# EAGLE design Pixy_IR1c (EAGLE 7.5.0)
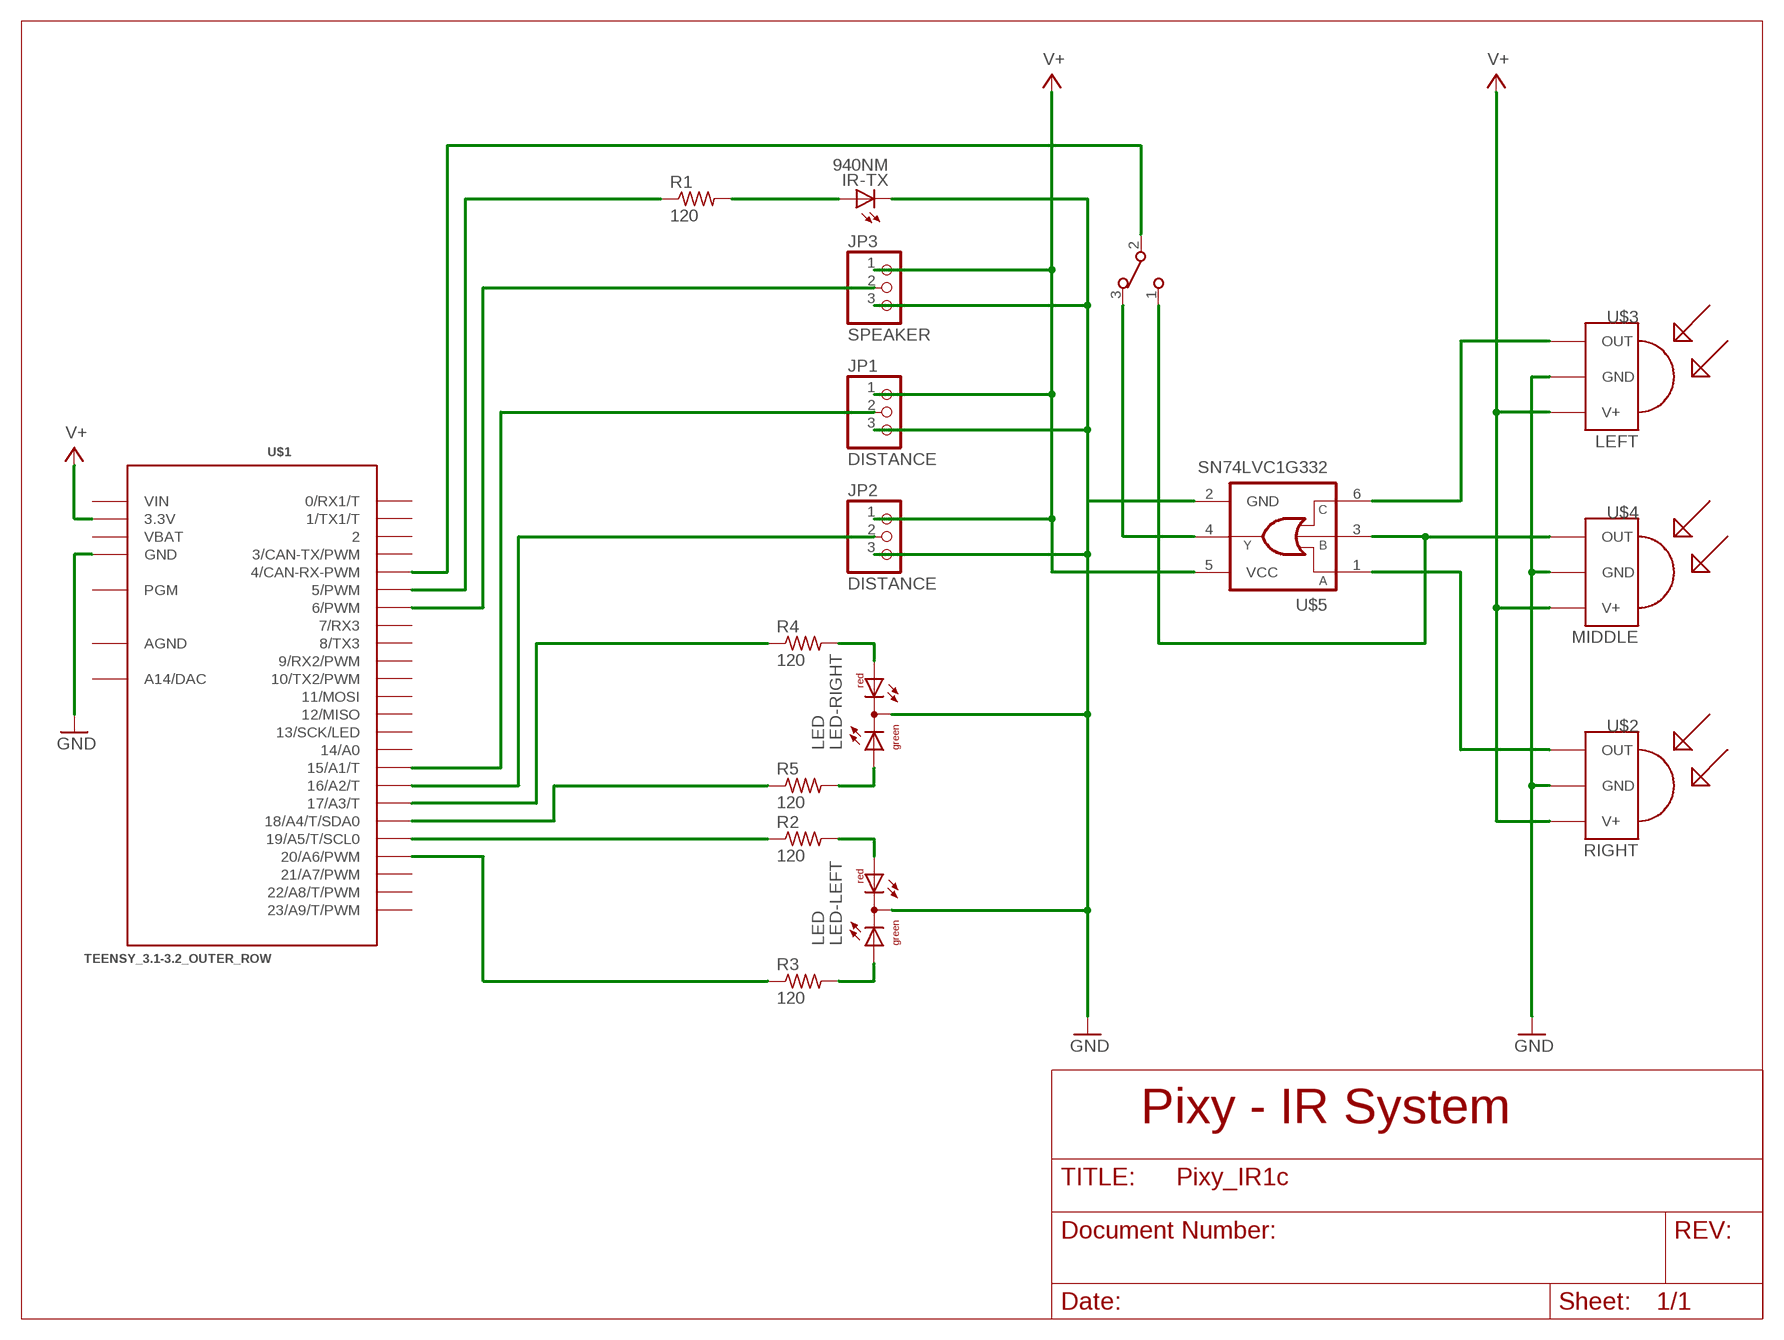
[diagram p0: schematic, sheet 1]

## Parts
IR-TX  940NM  LED5MM  [LED5MM]
JP1  DISTANCE  PINHD-1X3  [1X03]
JP2  DISTANCE  PINHD-1X3  [1X03]
JP3  SPEAKER  PINHD-1X3  [1X03]
LED-LEFT  LED  DUOLED-RG-C  [DUOLED-C-5MM]
LED-RIGHT  LED  DUOLED-RG-C  [DUOLED-C-5MM]
R1  120  R-US_R1206  [R1206]
R2  120  R-US_R1206  [R1206]
R3  120  R-US_R1206  [R1206]
R4  120  R-US_R1206  [R1206]
R5  120  R-US_R1206  [R1206]
SW1  CAS-120CAS-120B1  [CAS-120B1]
U$1  TEENSY_3.1-3.2_OUTER_ROW  [TEENSY_3.0-3.2&LC_OUTER_ROW]
U$2  RIGHT  TSOP3X  [TSOP18XX]
U$3  LEFT  TSOP3X  [TSOP18XX]
U$4  MIDDLE  TSOP3X  [TSOP18XX]
U$5  SN74LVC1G332  [SC70-6]

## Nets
GND: IR-TX.K(C) JP1.3 JP2.3 JP3.3 LED-LEFT.C LED-RIGHT.C U$1.GND U$1.GND1(GND) U$2.GND U$3.GND U$4.GND U$5.2(GND)
N$1: R2.1 U$1.19/A5(19/A5/T/SCL0)
N$2: R5.1 U$1.18/A4(18/A4/T/SDA0)
N$3: LED-RIGHT.AR R4.2
N$4: LED-RIGHT.AX(AG) R5.2
N$5: LED-LEFT.AR R2.2
N$6: LED-LEFT.AX(AG) R3.2
N$7: JP3.2 U$1.6(6/PWM)
N$8: R1.1 U$1.5(5/PWM)
N$9: R4.1 U$1.17/A3(17/A3/T)
N$10: R3.1 U$1.20/A6(20/A6/PWM)
N$11: JP1.2 U$1.15/A1(15/A1/T)
N$12: IR-TX.A R1.2
N$13: JP2.2 U$1.16/A2(16/A2/T)
N$14: SW1.2 U$1.4(4/CAN-RX-PWM)
N$15: SW1.3 U$5.4(Y)
N$16: SW1.1 U$4.OUT U$5.3(B)
N$17: U$3.OUT U$5.6(C)
N$18: U$2.OUT U$5.1(A)
V+: JP1.1 JP2.1 JP3.1 U$1.3.3V U$1.3.3V1(3.3V) U$2.VCC(V+) U$3.VCC(V+) U$4.VCC(V+) U$5.5(VCC)
Unconnected: U$1.0(0/RX1/T) U$1.1(1/TX1/T) U$1.2 U$1.3(3/CAN-TX/PWM) U$1.7(7/RX3) U$1.8(8/TX3) U$1.9(9/RX2/PWM) U$1.10(10/TX2/PWM) U$1.11(11/MOSI) U$1.12(12/MISO) U$1.13(13/SCK/LED) U$1.14/A0 U$1.21/A7(21/A7/PWM) U$1.22/A8(22/A8/T/PWM) U$1.23/A9(23/A9/T/PWM) U$1.PGM U$1.RESET/DAC(A14/DAC)

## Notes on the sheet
- Pixy - IR System

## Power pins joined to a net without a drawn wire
AGND: U$1.AGND
VBAT: U$1.VBAT
VIN: U$1.VIN

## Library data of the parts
IR-TX = led:LED: LED
JP1-JP3 = pinhead:PINHD-1X3: PIN HEADER
LED-LEFT LED-RIGHT = led:DUOLED-RG-C: DUO LED 2 colors (red/green), 5 mm, round, common Cathode www.ligitek.com or other producers.
R1-R5 = resistor:R-US_: RESISTOR, American symbol
SW1 = Switch2:CAS-120: CAS-120 surface mount type slide switch Producted by COPAL ELECTRONICS Store Information : Digi-Key : http://search.digikey.com/scripts/DkSearch/dksus.dll?Detail&name=CAS120GCT-ND
U$1 = Teensy_3_and_LC_Series_Boards_v1.4:TEENSY_3.1-3.2_OUTER_ROW: Footprint for Teensy 3.1 or 3.2 board using all pin connections on the outer perimeter
U$2-U$4 = _Loper:TSOP3X: IR Receiver and Demodulator
U$5 = 74LV:SN74LVC1G332: OR GATE 3-INPUT

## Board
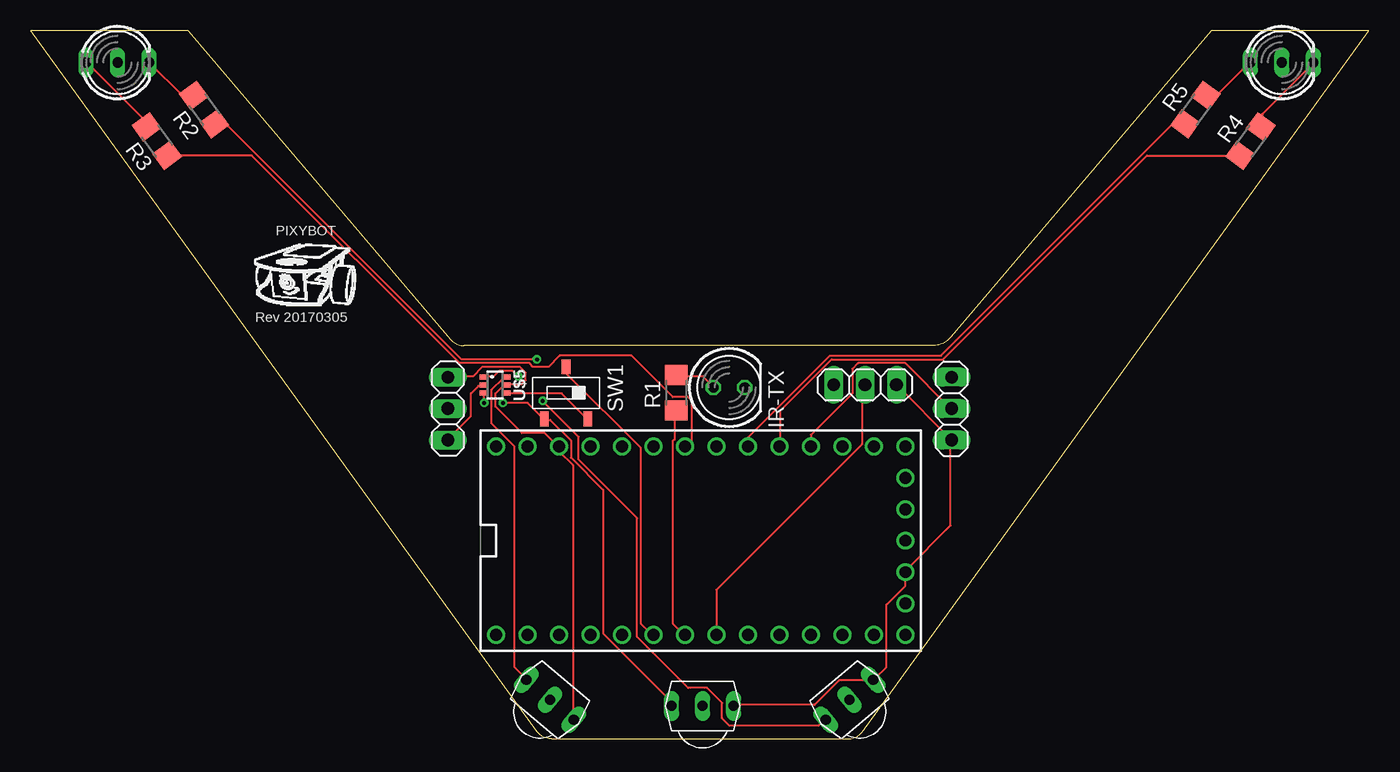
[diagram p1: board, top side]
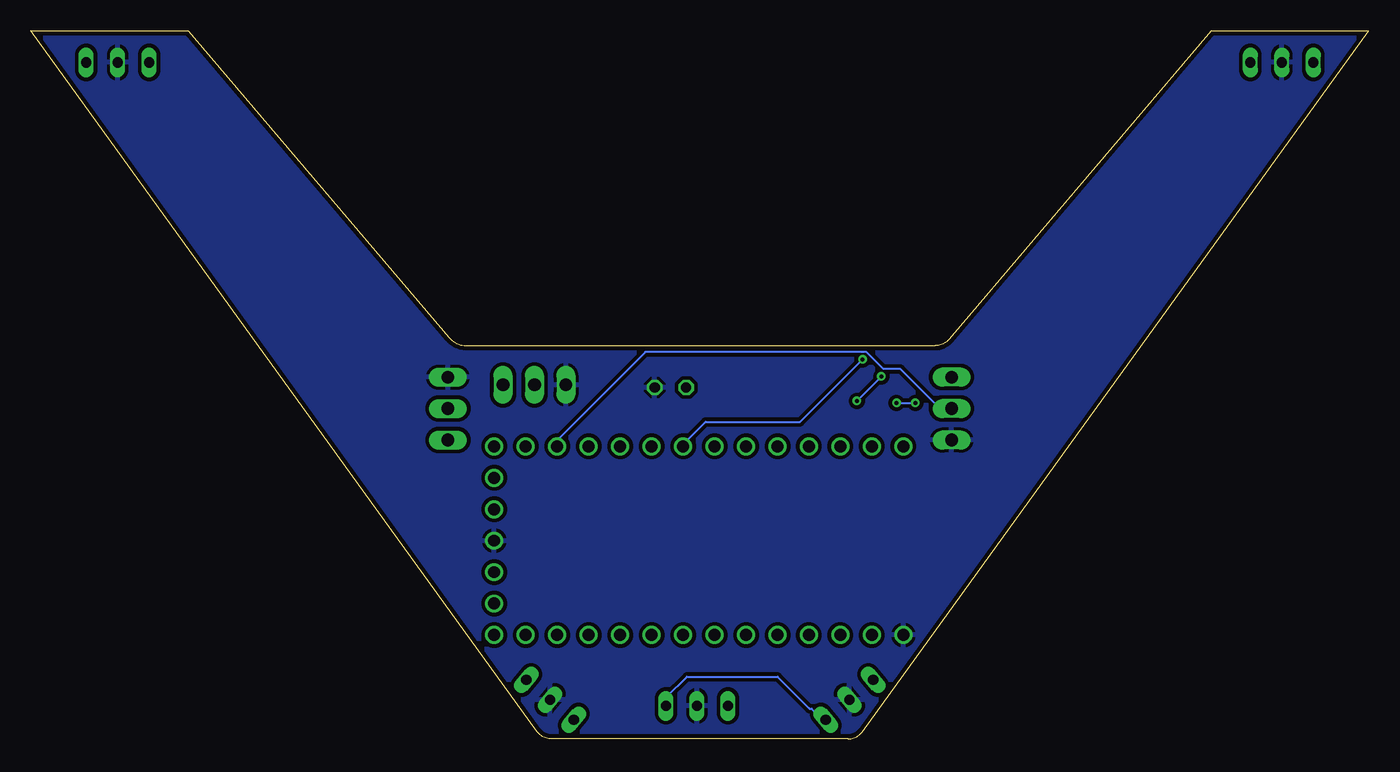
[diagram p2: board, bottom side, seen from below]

Size 107.95 x 57.15 mm. Coordinates in mm from the lower left corner, seen from the top.
Outline: 42,0 65.95,0 arc54 67.1,0.59 107.95,57.15 95.25,57.15 74.2,32.38 arc-50 72.83,31.75 34.95,31.75 arc-50 33.87,32.25 12.7,57.15 0,57.15 40.85,0.59 arc54 42,0
Copper layers (1*16): Top 0.0356mm / dielectric 1.5011mm / Bottom 0.0356mm
Design rules "oshpark-2layer": minimum track width 6mil, minimum drill 13mil, track to track 6mil, track to pad 6mil, pad to pad 6mil, via to via 6mil, smd to smd 6mil, copper to edge 15mil, drill to drill 6mil, minimum pad ring 7mil, minimum via ring 7mil, stop-mask expansion 2.5mil, vias tented up to drill 0mil, thermal gap 10mil

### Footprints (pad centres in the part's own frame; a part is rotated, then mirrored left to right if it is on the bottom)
LED5MM = drill 0.813 octagon: A -1.27,0; K 1.27,0
1X03 = drill 1.016 long: 1 -2.54,0; 2 0,0; 3 2.54,0
DUOLED-C-5MM = drill 0.813 long: AR 2.54,0; AX -2.54,0; C 0,0
R1206 = smd 1.6 x 1.803: 1 -1.422,0; 2 1.422,0
CAS-120B1 = smd 0.7 x 1.2: 1 -1.75,-2.1; 2 0,2.1; 3 1.75,-2.1
TEENSY_3.0-3.2&LC_OUTER_ROW = drill 0.965: 0 -7.62,13.97; 1 -7.62,11.43; 2 -7.62,8.89; 3 -7.62,6.35; 3.3V 7.62,11.43; 3.3V1 -2.54,-16.51; 4 -7.62,3.81; 5 -7.62,1.27; 6 -7.62,-1.27; 7 -7.62,-3.81; 8 -7.62,-6.35; 9 -7.62,-8.89; 10 -7.62,-11.43; 11 -7.62,-13.97; 12 -7.62,-16.51; 13 7.62,-16.51; 14/A0 7.62,-13.97; 15/A1 7.62,-11.43; 16/A2 7.62,-8.89; 17/A3 7.62,-6.35; 18/A4 7.62,-3.81; 19/A5 7.62,-1.27; 20/A6 7.62,1.27; 21/A7 7.62,3.81; 22/A8 7.62,6.35; 23/A9 7.62,8.89; AGND 7.62,13.97; GND -7.62,16.51; GND1 0,-16.51; PGM 2.54,-16.51; RESET/DAC 5.08,-16.51; VBAT -5.08,-16.51; VIN 7.62,16.51
TSOP18XX = drill 0.813 long: GND -0.001,-0.027; OUT -2.501,-0.027; VCC 2.499,-0.027
SC70-6 = smd 0.4 x 0.6: 1 -0.65,-0.95; 2 0,-0.95; 3 0.65,-0.95; 4 0.65,0.95; 5 0,0.95; 6 -0.65,0.95

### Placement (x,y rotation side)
IR-TX  56.34,28.37 0 top
JP1  33.66,26.67 270 top
JP2  74.3,26.67 90 top
JP3  67.31,28.57 180 top
LED-LEFT  6.99,54.61 0 top
LED-RIGHT  100.97,54.61 0 top
R1  52.07,27.94 90 top
R2  13.97,50.8 126 top
R3  10.16,48.26 126 top
R4  98.42,48.26 54 top
R5  93.98,50.8 54 top
SW1  43.18,27.94 0 top
U$1  54.05,16 90 top
U$2  66.04,3.17 40 top
U$3  41.91,3.17 320 top
U$4  54.2,2.69 0 top
U$5  37.47,28.57 270 top

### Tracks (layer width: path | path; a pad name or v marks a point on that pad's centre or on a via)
GND
  Top 0.152: U$5.2 36.42,28.5 36.12,28.5 35.51,27.89 35.51,26.06 33.68,24.23 JP1.3
  pour Bottom (isolate 0.305): 0,57.15 12.7,57.15 34.29,31.75 73.66,31.75 95.25,57.15 107.95,57.15 66.67,0 41.27,0
N$1  (via drill 0.33)
  Top 0.152: v40.84,30.63 34.75,30.63 15.85,49.53 14.94,49.53 R2.1
  Bottom 0.152: v40.84,30.63 45.87,25.6 53.49,25.6 55.32,23.77 U$1.19/A5
N$2
  Top 0.152: R5.1 93.12,49.53 92.05,49.53 73.46,30.94 64.47,30.94 57.91,24.38 57.91,23.62 U$1.18/A4
N$3
  Top 0.152: R4.2 99.36,49.53 99.36,50.44 103.48,54.56 LED-RIGHT.AR
N$4
  Top 0.152: R5.2 94.94,51.97 95.71,51.97 98.3,54.56 LED-RIGHT.AX
N$5
  Top 0.152: R2.2 13.11,51.97 12.19,51.97 9.6,54.56 LED-LEFT.AR
N$6
  Top 0.152: R3.2 9.3,49.53 9.3,49.84 4.57,54.56 LED-LEFT.AX
N$7
  Top 0.152: U$1.6 55.32,12.04 67.06,23.77 67.06,28.35 67.21,28.5 JP3.2
N$8
  Top 0.152: R1.1 51.97,26.52 51.97,24.23 51.82,24.08 51.82,9.3 52.73,8.38 U$1.5
N$9
  Top 0.152: R4.1 97.54,47.09 90.07,47.09 73.61,30.63 64.62,30.63 60.5,26.52 60.5,23.62 U$1.17/A3
N$10
  Top 0.152: R3.1 11.12,47.09 17.83,47.09 34.59,30.33 40.23,30.33 40.54,30.02 41.76,30.02 42.67,30.94 48.46,30.94 51.82,27.58 53.03,27.58 53.34,27.28 53.34,24.08 52.88,23.62 U$1.20/A6
N$11
  Bottom 0.152: JP1.2 34.59,26.67 37.8,29.87 39.17,29.87 40.54,31.24 58.37,31.24 65.38,24.23 65.38,23.62 U$1.15/A1
N$12
  Top 0.152: R1.2 52.12,29.26 54.25,29.26 55.02,28.5 IR-TX.A
N$13
  Top 0.152: U$1.16/A2 62.94,24.54 66.29,27.89 66.29,29.87 66.75,30.33 70.56,30.33 74.22,26.67 JP2.2
N$14
  Top 0.152: SW1.2 43.28,30.02 43.28,29.41 49.23,23.47 49.23,9.3 50.14,8.38 U$1.4
N$15
  Top 0.152: U$5.4 38.56,27.89 42.82,27.89 44.81,25.91 SW1.3
N$16  (via drill 0.33)
  Top 0.152: v36.58,27.13 36.58,27.89 U$5.3 | v38.1,27.13 40.08,27.13 41.3,25.91 SW1.1 41.45,25.76 41.91,25.76 43.59,24.08 43.59,22.71 46.18,20.12 46.18,8.53 51.66,3.05 51.66,2.74 U$4.OUT
  Bottom 0.152: v38.1,27.13 v36.58,27.13
N$17
  Top 0.152: U$5.6 38.41,29.11 38.1,29.11 37.19,28.19 37.19,25.45 39.01,23.62 39.01,5.79 39.93,4.88 U$3.OUT
N$18  (via drill 0.33)
  Top 0.152: v39.32,29.26 38.86,29.72 37.8,29.72 37.34,29.26 36.58,29.26 U$5.1 | v41.3,27.28 44.2,24.38 44.2,22.55 48.92,17.83 48.92,8.23 53.03,4.12 54.56,4.12 55.78,2.9 55.78,1.68 56.39,1.07 63.55,1.07 64.01,1.52 U$2.OUT
  Bottom 0.152: v41.3,27.28 v39.32,29.26
V+
  Top 0.152: U$3.VCC 43.74,1.68 43.74,22.1 42.67,23.16 42.67,23.62 U$1.3.3V 42.52,23.62 41.45,24.69 39.62,24.69 37.49,26.82 37.49,27.89 38.1,28.5 38.41,28.5 U$5.5 38.56,28.65 39.62,28.65 39.93,28.96 39.93,29.57 39.47,30.02 36.42,30.02 35.66,29.26 33.68,29.26 JP1.1 | JP3.1 69.95,28.5 74.22,24.23 JP2.1 74.22,24.08 74.22,17.22 70.56,13.56 U$1.3.3V1 70.56,12.34 69.04,10.82 69.04,5.79 68.12,4.88 U$2.VCC 67.97,4.72 65.23,4.72 63.25,2.74 56.84,2.74 U$4.VCC
  Bottom 0.152: U$3.VCC 43.89,1.68 44.2,1.68 44.96,2.44 45.11,2.44 47.7,5.03 55.02,5.03 56.69,3.35 56.69,2.74 U$4.VCC

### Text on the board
tPlace: PIXYBOT | Rev 20170305

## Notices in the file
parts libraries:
74LV: Copyright (C) 2008, Bob Starr
